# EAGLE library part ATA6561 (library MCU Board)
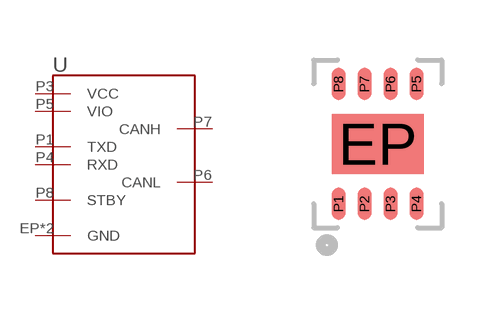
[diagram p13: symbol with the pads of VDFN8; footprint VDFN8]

Designator prefix U

## ATA6561  [VDFN8]
EP  GND
P1  TXD
P2  GND
P3  VCC
P4  RXD
P5  VIO
P6  CANL
P7  CANH
P8  STBY

## Footprint VDFN8 (pad centres in mm)
smd 2.3 x 1.5: EP 0,0
smd 0.35 x 0.8: P1 -0.975,-1.5; P2 -0.325,-1.5; P3 0.325,-1.5; P4 0.975,-1.5; P5 0.975,1.5; P6 0.325,1.5; P7 -0.325,1.5; P8 -0.975,1.5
